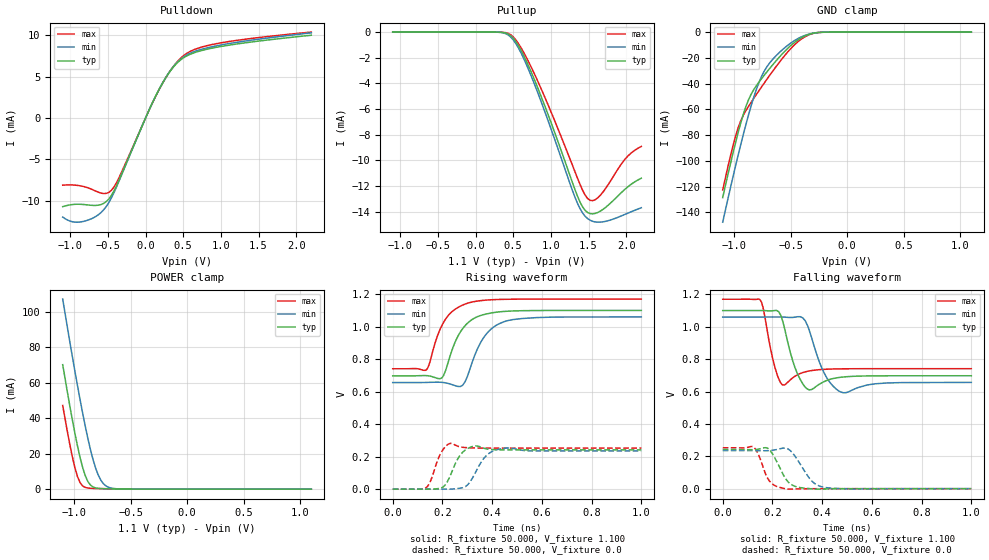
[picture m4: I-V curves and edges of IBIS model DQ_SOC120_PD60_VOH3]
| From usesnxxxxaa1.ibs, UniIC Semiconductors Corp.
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|   Model DQ_SOC120_PD60_VOH3
[Model] DQ_SOC120_PD60_VOH3
Model_type I/O
Polarity   Non-Inverting
Enable   Active-High
Vinl =  0.113V
Vinh =  0.253V
Vmeas =  0.183V
Rref =  50.000
Vref =  0.183V
C_comp   1.110pF   1.087pF   1.118pF
[Model Spec]
Vinh   0.253V   0.247V   0.265V
Vinl   0.113V   0.107V   0.125V
Vmeas   0.183V   NA   NA
Vref   0.183V   NA   NA
Rref   50.000   NA   NA
[Temperature Range]   25.000   0.125k   -40.000
[Voltage Range]   1.100V   1.060V   1.170V
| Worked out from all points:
|   slope of the pulldown table from 0 to 0.165 V, typ, clamps not added: 51.4 ohm
|   GND clamp passes 1 mA (typ) near -0.30 V on its own axis
|   POWER clamp passes 1 mA (typ) near -0.82 V on its own axis
|   rising waveform, R_fixture 50.000, V_fixture 1.100: 20-80 % time 77ps typ, 81.4ps min, 75.6ps max; typ from 0.697 V to 1.1 V
|   rising waveform, R_fixture 50.000, V_fixture 0.0: 20-80 % time 43.9ps typ, 53.9ps min, 35ps max; typ from 0 V to 0.242 V
|   falling waveform, R_fixture 50.000, V_fixture 1.100: 20-80 % time 40.2ps typ, 53.2ps min, 31ps max; typ from 1.1 V to 0.697 V
|   falling waveform, R_fixture 50.000, V_fixture 0.0: 20-80 % time 51.5ps typ, 62.1ps min, 40.6ps max; typ from 0.242 V to 0 V
[Pulldown]
|Voltage   I(typ)   I(min)   I(max)
-1.1V     -10.75mA   -12.01mA   -8.142mA
-930mV    -10.46mA   -12.63mA   -8.143mA
-726mV    -10.58mA   -12.24mA   -8.599mA
-556mV    -10.35mA   -11.12mA   -9.157mA
-454mV    -9.387mA   -9.688mA   -8.773mA
-352mV    -7.516mA   -7.642mA   -7.222mA
158mV     3.086mA    3.099mA    3.057mA
328mV     5.681mA    5.734mA    5.724mA
498mV     7.257mA    7.365mA    7.504mA
668mV     7.97mA     8.112mA    8.363mA
940mV     8.561mA    8.737mA    9mA
2.2V      10.02mA    10.31mA    10.4mA
[Pullup]
|Voltage   I(typ)   I(min)   I(max)
-1.1V     -58.82pA   9.882nA    0A
432mV     -148.6uA   -221.4uA   -100.6uA
568mV     -1.047mA   -1.224mA   -888.8uA
738mV     -3.104mA   -3.412mA   -2.724mA
976mV     -6.642mA   -7.121mA   -5.859mA
1.316V    -12.21mA   -12.81mA   -10.83mA
1.418V    -13.59mA   -14.07mA   -12.29mA
1.486V    -14.05mA   -14.52mA   -12.96mA
1.554V    -14.16mA   -14.74mA   -13.13mA
1.622V    -14.05mA   -14.81mA   -12.91mA
1.996V    -12.18mA   -14.16mA   -9.815mA
2.2V      -11.38mA   -13.68mA   -8.909mA
[GND_clamp]
|Voltage   I(typ)   I(min)   I(max)
-1.1V     -128.5mA   -147.6mA   -122.6mA
-1.008V   -93.62mA   -112mA     -87.95mA
-962mV    -77.6mA    -95.05mA   -73.96mA
-893mV    -57.36mA   -71.21mA   -60.7mA
-847mV    -48.01mA   -56.81mA   -54.36mA
-801mV    -41.47mA   -44.23mA   -48.33mA
-755mV    -36.02mA   -34.19mA   -42.41mA
-709mV    -30.9mA    -26.94mA   -36.63mA
-525mV    -12.67mA   -10.3mA    -15.49mA
-387mV    -3.615mA   -3.065mA   -4.419mA
-249mV    -281uA     -330.6uA   -301.3uA
1.1V      0A         0A         0A
[POWER_clamp]
|Voltage   I(typ)   I(min)   I(max)
-1.1V     70.27mA    107.3mA    47.25mA
-1.039V   47.68mA    83.93mA    25.86mA
-993mV    31.88mA    66.94mA    12.35mA
-970mV    24.65mA    58.72mA    7.262mA
-947mV    18.06mA    50.74mA    3.761mA
-901mV    7.73mA     35.71mA    987.1uA
-855mV    2.348mA    22.46mA    514uA
-809mV    697.3uA    11.94mA    396.5uA
-763mV    321uA      5.097mA    322.7uA
-717mV    213.8uA    1.813mA    258.1uA
-556mV    65.24uA    79.15uA    81.64uA
1.1V      0A         0A         0A
[Ramp]
| variable   typ   min   max
dV/dt_r   0.145/43.972p   0.141/54.973p   0.152/35.407p
dV/dt_f   0.242/40.563p   0.242/54.206p   0.257/31.064p
R_load = 50.000
[Rising Waveform]
R_fixture= 50.000
V_fixture= 1.100
V_fixture_min= 1.060
V_fixture_max= 1.170
|time   V(typ)   V(min)   V(max)
0s        697.4mV    656.2mV    741mV
136ps     698.6mV    656.8mV    735.2mV
198ps     685.5mV    657.3mV    1.008V
230ps     816.3mV    647.6mV    1.08V
272ps     966.9mV    631.7mV    1.126V
291ps     1.006V     660.6mV    1.139V
309ps     1.032V     732mV      1.148V
366ps     1.074V     933.4mV    1.162V
456ps     1.095V     1.035V     1.169V
1ns       1.1V       1.06V      1.17V
[Rising Waveform]
R_fixture= 50.000
V_fixture= 0.0
V_fixture_min= 0.0
V_fixture_max= 0.0
|time   V(typ)   V(min)   V(max)
0s        2.218uV    17.94uV    414.7nV
139ps     -72.22uV   -2.896uV   15.05mV
195ps     7.993mV    -119.8uV   225.5mV
232ps     85.05mV    80.99uV    281.8mV
262ps     187.5mV    4.29mV     264mV
302ps     250.7mV    27.47mV    255mV
335ps     265.7mV    108.8mV    253.3mV
377ps     247.7mV    207.2mV    252.8mV
436ps     241.9mV    248.7mV    252.6mV
1ns       241.7mV    235.4mV    252.6mV
[Falling Waveform]
R_fixture= 50.000
V_fixture= 1.100
V_fixture_min= 1.060
V_fixture_max= 1.170
|time   V(typ)   V(min)   V(max)
0s        1.1V       1.06V      1.17V
150ps     1.1V       1.06V      1.167V
212ps     1.101V     1.06V      738.3mV
240ps     1.041V     1.06V      640.9mV
291ps     746.8mV    1.059V     694.5mV
322ps     648.1mV    1.055V     716.9mV
347ps     610.4mV    983.6mV    726.7mV
407ps     660.5mV    717.3mV    736.9mV
474ps     688mV      597.5mV    740mV
1ns       697.4mV    656.2mV    741mV
[Falling Waveform]
R_fixture= 50.000
V_fixture= 0.0
V_fixture_min= 0.0
V_fixture_max= 0.0
|time   V(typ)   V(min)   V(max)
0s        241.7mV    235.4mV    252.6mV
124ps     240.9mV    235.1mV    257.2mV
145ps     244.5mV    234.6mV    205.7mV
182ps     248.7mV    234.8mV    61.39mV
207ps     196.8mV    238.9mV    21.2mV
254ps     59.22mV    249.8mV    -603.3uV
282ps     20.38mV    218.8mV    -2.553mV
358ps     -900uV     47.7mV     -171.8uV
408ps     -2.204mV   8.482mV    -24.12uV
1ns       3.636uV    20.69uV    2.458uV
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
